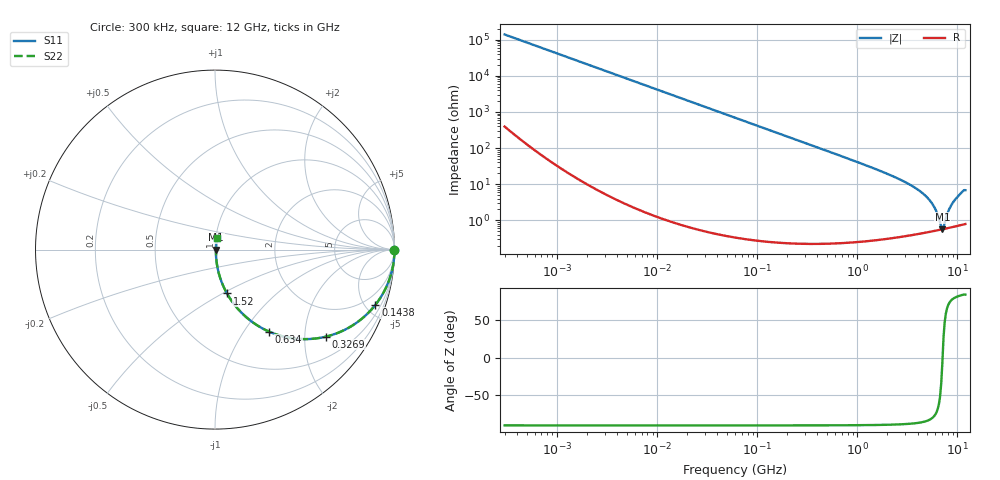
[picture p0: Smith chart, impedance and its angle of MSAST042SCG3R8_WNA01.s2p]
! MSAST042SCG3R8_WNA01  S-PARAMETER MODEL  ( General Type )
! Model Generated by TAIYO YUDEN Corporation (http://www.ty-top.com)
! Version 1.0
! TAIYO YUDEN Control No. 150820
! Copyright(c) 2015 TAIYO YUDEN CO.,LTD. All Rights Reserved.
! Product Description (link to TY-COMPAS)
! https://ds.yuden.co.jp/TYCOMPAS/or/detail?pn=MSAST042SCG3R8BWNA01&u=M
! Products Name : Multilayer Ceramic Capacitors
! Characteristics :
!  Capacitance : 3.8 pF , Rated Voltage : 25V , TCC : CG / C0G
!  Case Size : 0.4 x 0.2 / 0.016 x 0.008 [mm/inch] , Thickness : 0.2 / 0.008 [mm/inch]
!  (Conditions: Temperature = 25 degC , DC Bias Current/Voltage = 0A / 0V)
! External Node Assignments :
!  1  o---| |---o  2
! GND o---------o GND
! Frequency Range : 0.3MHz  -  12000MHz  [ 401 STEP ]
# MHz S RI R 50
! Freq[MHz].  S11 Real  S11 Imag  S21 Real  S21 Imag  S12 Real  S12 Imag  S22 Real  S22 Imag
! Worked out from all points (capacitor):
!   401 points, 300 kHz to 12 GHz, reference 50 ohm
!   read as one part in series: C = 3.81 pF near 316.3 kHz
!   lowest |Z| = 568 mohm at 7.064 GHz (marker M1)
!   series resonance near 7.102 GHz, so ESL is about 130 pH
!   S11 on the Smith chart (normalised r, x): 300 kHz: open; 143.8 MHz: 1.00, -5.80; 326.9 MHz: 1.00, -2.55; 634 MHz: 1.00, -1.31; 1.52 GHz: 1.01, -0.52; 12 GHz: 1.02, +0.14
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0.3  1 -0.000719  2.54e-06 0.000719  2.54e-06 0.000719  1 -0.000719
1.769972  1 -0.00424  2.01e-05 0.00424  2.01e-05 0.00424  1 -0.00424
10.44266  0.9994 -0.025  0.000633 0.025  0.000633 0.025  0.9994 -0.025
60  0.9797 -0.1408  0.0203 0.1408  0.0203 0.1408  0.9797 -0.1408
143.8206  0.8936 -0.3079  0.1064 0.3079  0.1064 0.3079  0.8936 -0.3079
326.9496  0.6186 -0.4849  0.3814 0.4849  0.3814 0.4849  0.6186 -0.4849
353.9943  0.5804 -0.4926  0.4196 0.4926  0.4196 0.4926  0.5804 -0.4926
634.0297  0.2997 -0.4564  0.7003 0.4564  0.7003 0.4564  0.2997 -0.4564
968.706  0.1532 -0.3573  0.8468 0.3573  0.8468 0.3573  0.1532 -0.3573
1519.776  0.0666 -0.244  0.9334 0.244  0.9334 0.244  0.0666 -0.244
2088.533  0.0351 -0.1757  0.9649 0.1757  0.9649 0.1757  0.0351 -0.1757
3454.93  0.0122 -0.0908  0.9878 0.0908  0.9878 0.0908  0.0122 -0.0908
4747.894  0.00683 -0.0481  0.9932 0.0481  0.9932 0.0481  0.00683 -0.0481
5715.274  0.00562 -0.0255  0.9944 0.0255  0.9944 0.0255  0.00562 -0.0255
6188.031  0.00546 -0.0162  0.9945 0.0162  0.9945 0.0162  0.00546 -0.0162
6699.894  0.00548 -0.00687  0.9945 0.00687  0.9945 0.00687  0.00548 -0.00687
7064.448  0.00561 -0.000695  0.9944 0.000695  0.9944 0.000695  0.00561 -0.000695
7448.838  0.00582 0.00608  0.9942 -0.00608  0.9942 -0.00608  0.00582 0.00608
8281.503  0.00654 0.0193  0.9935 -0.0193  0.9935 -0.0193  0.00654 0.0193
8966.534  0.00734 0.0293  0.9927 -0.0293  0.9927 -0.0293  0.00734 0.0293
10793.46  0.0103 0.0544  0.9897 -0.0544  0.9897 -0.0544  0.0103 0.0544
12000  0.0123 0.0664  0.9877 -0.0664  0.9877 -0.0664  0.0123 0.0664
